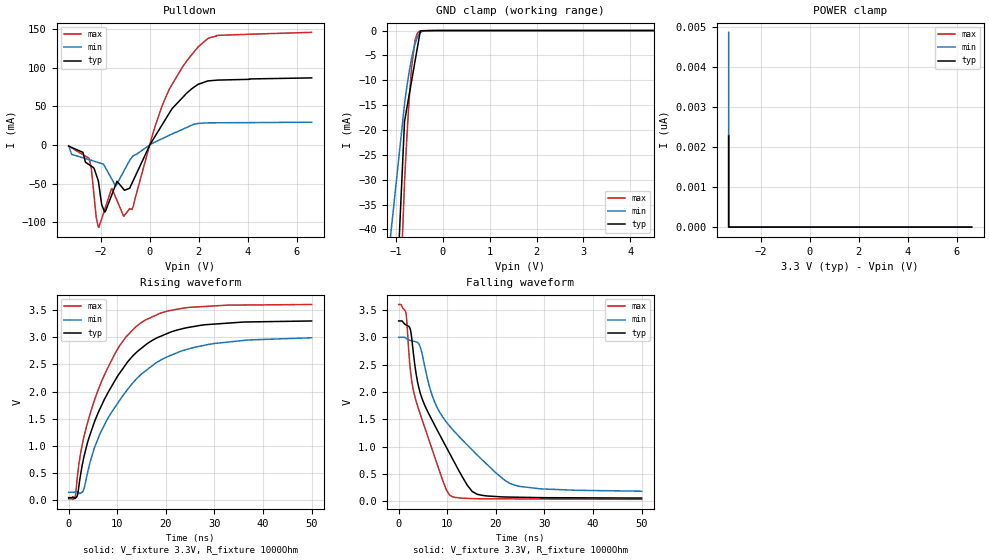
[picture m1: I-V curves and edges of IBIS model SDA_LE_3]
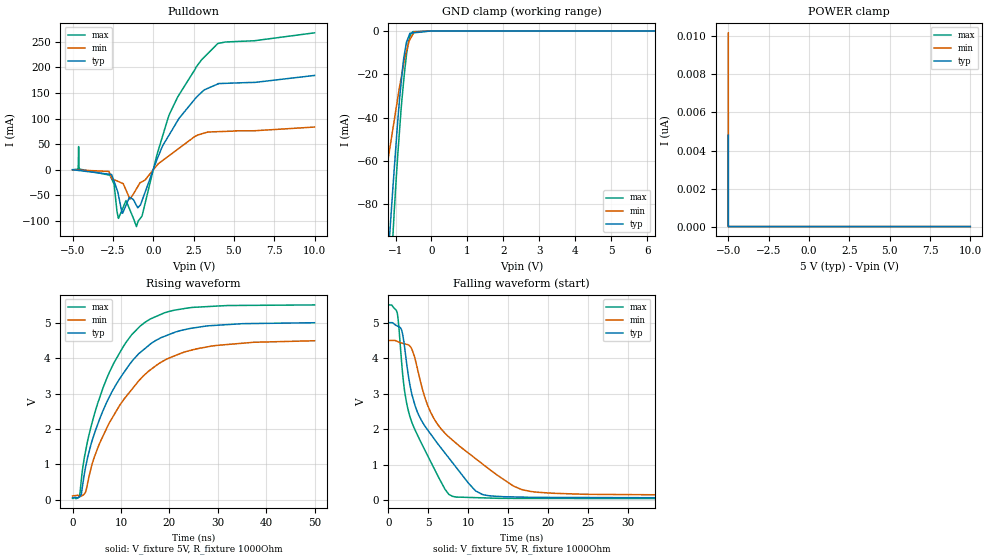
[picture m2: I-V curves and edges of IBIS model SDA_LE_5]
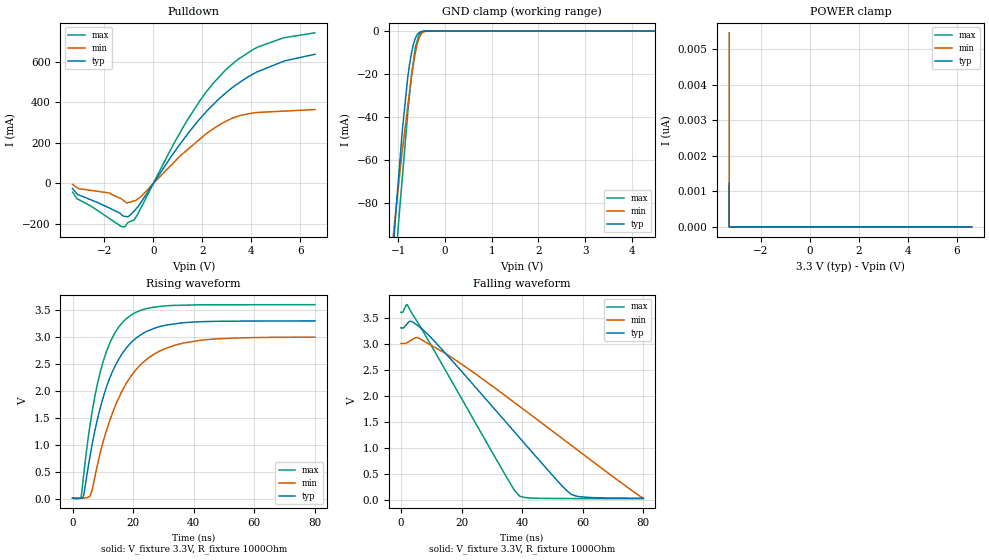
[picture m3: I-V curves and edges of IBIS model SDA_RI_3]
| Texas Instruments Incorporated
| Low-Power Bidirectional I2C Isolators
| Marketing part#   Voltage Range   Package-type   #pins/pkg drawing
| ISO1540D   3V-5.5V   SOIC   8-pin D
[IBIS Ver]   4.1
[File name]   iso1540.ibs
[File Rev]   1.0
[Date]   06/21/2012
[Source]   TIspiceD simulations
   Texas Instruments Incorporated.
   Analog eLab Design Center, HPA
   12500 TI Blvd
   Dallas, TX -75243
   For Support e-mail: elab_scm_ibis@list.ti.com
[Notes]   Revision History:
   Rev 1.0: 06/21/2012
   - C_comp although listed in numerical order of value are
   obtained from varying PVT conditions.
   For PVT conditions for each specific value, refer to the
   buffer description under respective [Model].
   IBIS model user is responsible for using appropriate
   C_comp to simulate for Signal Integrity.
   - IBIS model matched to TISPICED simulations
   - Pulldown data is non-monotonic, reflects circuit behavior
[Disclaimer] This model is designed as an aid for customers of Texas Instruments.
 TI and its licensors and suppliers make no warranties, either expressed
 or implied, with respect to this  model, including the warranties of
 merchantability or fitness for a particular purpose.
 The model is provided solely on an "as is" basis. The entire risk as to
 its quality and performance is with the customer.
[Copyright] (C)Copyright 2012 Texas Instruments Incorporated.
   All rights reserved.
|   Component ISO1540D
[Component]   ISO1540D
[Manufacturer]  Texas Instruments Incorporated
[Package]   |SOIC (D) 8-pin
|   typ   min   max
R_pkg   0.06626   0.03167   0.11324
L_pkg   2.49942nH   2.25405nH   2.79138nH
C_pkg   0.41610pF   0.38404pF   0.69535pF
[Pin]   signal_name   model_name   R_pin   L_pin   C_pin
1   VCC1   POWER   0.03718  2.27597n  0.43076p
2   SDA1   SDA_LE   0.09214  2.47816n  0.38404p
3   SCL1   SDA_LE   0.11324  2.79138n  0.40143p
4   GND1   GND   0.03348  2.51166n  0.69535p
5   GND2   GND   0.03167  2.53947n  0.67094p
6   SCL2   SDA_RI   0.09215  2.48718n  0.38609p
7   SDA2   SDA_RI   0.11323  2.77707n  0.39917p
8   VCC2   POWER   0.04038  2.25405n  0.46007p
[Model Selector] SDA_LE
SDA_LE_3   SDA I/O left side model for 3.0V - 3.6V
SDA_LE_5   SDA I/O left side model for 4.5V - 5.5V
[Model Selector] SDA_RI
SDA_RI_3   SDA I/O right side model for 3.0V - 3.6V
SDA_RI_5   SDA I/O right side model for 4.5V - 5.5V
| Models and submodels in the file (4): SDA_LE_3 (I/O_open_drain), SDA_LE_5 (I/O_open_drain), SDA_RI_3 (I/O_open_drain), SDA_RI_5 (I/O_open_drain)
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|   SDA Left 3.3V I/O Model
[Model]   SDA_LE_3
Model_type   I/O_open_drain
Polarity   Non-Inverting
Enable   Active-Low
Vinl = 0.5
Vinh = 2.52
Vmeas = 1.65
Vref = 1.65
Cref = 15pF
Rref = 1000
|   typ   min   max
|   (nom PVT)   (fast PVT)   (slow PVT)
C_comp   4.033p   3.367p   4.533p
|C_comp (High state)   4.033p   3.367p   4.533p
|C_comp (Low state)   5.596p   4.907p   5.983p
|PVT   Nom   Slow   Fast
[Voltage Range]   3.3   3   3.6
[Temperature Range]   27   136   -40
[Pullup Reference]   3.3   3   3.6
[Pulldown Reference]   -0   -0   -0
[Power Clamp Reference]   3.3   3   3.6
[GND Clamp Reference]   -0   -0   -0
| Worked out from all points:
|   slope of the pulldown table from 0 to 0.495 V, typ, clamps not added: 19.4 ohm
|   GND clamp passes 1 mA (typ) near -0.50 V on its own axis
|   falling waveform, V_fixture 3.3V, R_fixture 1000Ohm: 20-80 % time 8.4ns typ, 11.9ns min, 5.69ns max; typ from 3.3 V to 0.057 V
|   rising waveform, V_fixture 3.3V, R_fixture 1000Ohm: 20-80 % time 10.2ns typ, 12ns min, 8.59ns max; typ from 0.053 V to 3.3 V
[Pulldown]
|   Voltage   I(typ)   I(min)   I(max)
-3.3V     -1.441mA   -854.9uA   -1.481mA
-2.462V   -25.48mA   -19.01mA   -17.28mA
-2.095V   -46.15mA   -22.58mA   -105.6mA
-1.835V   -86.44mA   -27.36mA   -83.61mA
-1.533V   -63.51mA   -44.52mA   -56.4mA
-1.329V   -46.75mA   -49.98mA   -71.69mA
-1.058V   -57.16mA   -34.04mA   -92.04mA
-665.1mV  -45.59mA   -13.84mA   -78.65mA
800.2mV   41.16mA    12.55mA    72.1mA
1.984V    78.4mA     27.85mA    126.9mA
2.741V    83.72mA    28.65mA    141.4mA
6.6V      86.64mA    29.42mA    145.4mA
[GND Clamp]
|   Voltage   I(typ)   I(min)   I(max)
-3.3V     -815.4mA   -640mA     -971mA
-1.208V   -99.67mA   -49.74mA   -133.4mA
-1.091V   -75.48mA   -39.34mA   -97.6mA
-816.4mV  -18.3mA    -14.78mA   -30.7mA
-780mV    -16.34mA   -12.22mA   -23.92mA
-720.5mV  -13.12mA   -8.521mA   -14.39mA
-665.1mV  -10.12mA   -5.641mA   -7.366mA
-591.4mV  -6.144mA   -2.677mA   -1.944mA
-551.3mV  -3.973mA   -1.563mA   -734.8uA
-478.8mV  -55.54uA   -412.4uA   -98.93uA
-198.6mV  -17.66uA   -327nA     -154.7nA
6.6V      0A         0A         0A
[POWER Clamp]
|   Voltage   I(typ)   I(min)   I(max)
-3.3V     2.274nA    4.859nA    2.297nA
-3.3V     0A         0A         0A
-3.3V     0A         0A         0A
6.6V      0A         0A         0A
[Ramp]
R_load = 1000
|   typ   min   max
dV/dt_r   1.94673/1.02316e-08   1.70302/1.18334e-08   2.14001/8.58161e-09
dV/dt_f   1.9456/8.391e-09   1.69022/1.18691e-08   2.13948/5.67055e-09
[Falling Waveform]
V_fixture = 3.3V
V_fixture_min = 3V
V_fixture_max = 3.6V
R_fixture = 1000Ohm
C_fixture = 0F
|   Time   V(typ)   V(min)   V(max)
0s        3.3V       3V         3.6V
1.498ns   3.229V     2.986V     3.446V
2.486ns   3.108V     2.942V     2.34V
3.414ns   2.436V     2.921V     1.888V
5.316ns   1.765V     2.49V      1.361V
7.433ns   1.387V     1.809V     805.8mV
10.44ns   882.6mV    1.38V      115.5mV
15.14ns   177.9mV    938.5mV    48mV
23.88ns   73.47mV    293.4mV    42.9mV
50ns      57.34mV    183mV      34.2mV
[Rising Waveform]
V_fixture = 3.3V
V_fixture_min = 3V
V_fixture_max = 3.6V
R_fixture = 1000Ohm
C_fixture = 0F
|   Time   V(typ)   V(min)   V(max)
0s        52.63mV    150.1mV    32.79mV
1.366ns   41.87mV    157.1mV    77.54mV
1.856ns   113mV      153.4mV    486.1mV
2.88ns    687.9mV    157.4mV    1.06V
6.136ns   1.625V     1.156V     2.046V
9.812ns   2.245V     1.751V     2.744V
13.76ns   2.704V     2.214V     3.185V
18.88ns   3.014V     2.576V     3.44V
25.88ns   3.197V     2.813V     3.552V
50ns      3.297V     2.988V     3.599V
|   SDA Left 5V I/O Model
[Model]   SDA_LE_5
Model_type   I/O_open_drain
Polarity   Non-Inverting
Enable   Active-Low
Vinl = 0.5
Vinh = 3.85
Vmeas = 2.5
Vref = 2.5
Cref = 15pF
Rref = 1000
|   typ   min   max
|   (nom PVT)   (fast PVT)   (slow PVT)
C_comp   3.824p   3.201p   4.341p
|C_comp (ON state)   3.824p   3.201p   4.341p
|C_comp (OFF state)   4.090p   3.369p   4.747p
|PVT   Nom   Slow   Fast
[Voltage Range]   5   4.5   5.5
[Temperature Range]   27   136   -40
[Pullup Reference]   5   4.5   5.5
[Pulldown Reference]   -0   -0   -0
[Power Clamp Reference]   5   4.5   5.5
[GND Clamp Reference]   -0   -0   -0
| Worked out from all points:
|   slope of the pulldown table from 0 to 0.75 V, typ, clamps not added: 13.5 ohm
|   GND clamp passes 1 mA (typ) near -0.59 V on its own axis
|   falling waveform, V_fixture 5V, R_fixture 1000Ohm: 20-80 % time 5.86ns typ, 8.17ns min, 3.71ns max; typ from 5 V to 0.061 V
|   rising waveform, V_fixture 5V, R_fixture 1000Ohm: 20-80 % time 10ns typ, 11.6ns min, 8.51ns max; typ from 0.058 V to 5 V
[Pulldown]
|   Voltage   I(typ)   I(min)   I(max)
-5V       114.9uA    34.82uA    189.2uA
-4.66V    -1.19mA    -456.2uA   1.163mA
-4.624V   -1.328mA   -507.9uA   45.41mA
-4.584V   -1.482mA   -565.8uA   1.547mA
-2.677V   -8.802mA   -8.11mA    -10.73mA
-2.169V   -47.15mA   -22.82mA   -93.81mA
-1.93V    -84.92mA   -26.14mA   -78.43mA
-1.686V   -69.33mA   -39.6mA    -60.1mA
-1.039V   -69.58mA   -37.18mA   -111mA
1.024V    70.1mA     28.52mA    109.9mA
2.995V    151.3mA    70.22mA    214.8mA
10V       184.4mA    83.55mA    267.7mA
[GND Clamp]
|   Voltage   I(typ)   I(min)   I(max)
-5V       -1.078A    -841.4mA   -1.257A
-1.536V   -182.6mA   -122mA     -238.4mA
-1.234V   -111.6mA   -63.88mA   -147.4mA
-1.215V   -106.8mA   -60.09mA   -141mA
-1.108V   -80.87mA   -48.84mA   -105.3mA
-1.073V   -72.38mA   -45.15mA   -94.57mA
-911.4mV  -36.12mA   -28.15mA   -51.25mA
-767.8mV  -12.11mA   -14.79mA   -22.09mA
-695.2mV  -5.155mA   -9.331mA   -10.98mA
-638.6mV  -2.707mA   -5.775mA   -4.887mA
-516.2mV  -876.4uA   -1.491mA   -277.5uA
10V       0A         0A         0A
[POWER Clamp]
|   Voltage   I(typ)   I(min)   I(max)
-5V       4.793nA    10.19nA    5.967nA
-5V       0A         0A         0A
-5V       0A         0A         0A
10V       0A         0A         0A
[Ramp]
R_load = 1000
|   typ   min   max
dV/dt_r   2.96373/1.0022e-08   2.62546/1.15746e-08   3.27428/8.51231e-09
dV/dt_f   2.96329/5.82536e-09   2.62267/8.14594e-09   3.2739/3.70478e-09
[Falling Waveform]
V_fixture = 5V
V_fixture_min = 4.5V
V_fixture_max = 5.5V
R_fixture = 1000Ohm
C_fixture = 0F
|   Time   V(typ)   V(min)   V(max)
0s        5V         4.5V       5.5V
1.116ns   4.906V     4.473V     5.271V
1.99ns    4.392V     4.406V     3.159V
2.813ns   3.125V     4.308V     2.279V
3.802ns   2.399V     3.552V     1.764V
5.274ns   1.872V     2.489V     1.1V
8.039ns   1.056V     1.693V     109.3mV
11.79ns   160.4mV    1.021V     67.6mV
17.66ns   83.02mV    252.6mV    51.97mV
50ns      61.18mV    128.9mV    43.5mV
[Rising Waveform]
V_fixture = 5V
V_fixture_min = 4.5V
V_fixture_max = 5.5V
R_fixture = 1000Ohm
C_fixture = 0F
|   Time   V(typ)   V(min)   V(max)
0s        57.65mV    113mV      42.31mV
1.449ns   85.7mV     109.5mV    119.9mV
3.02ns    1.136V     406.6mV    1.605V
4.453ns   1.844V     1.19V      2.385V
6.324ns   2.525V     1.81V      3.171V
10.37ns   3.545V     2.791V     4.298V
13.98ns   4.158V     3.402V     4.904V
18.66ns   4.596V     3.913V     5.257V
25.66ns   4.864V     4.262V     5.436V
50ns      4.997V     4.489V     5.499V
|   SDA Right 3.3V I/O Model
[Model]   SDA_RI_3
Model_type   I/O_open_drain
Polarity   Non-Inverting
Enable   Active-Low
Vinl = 0.9
Vinh = 2.52
Vmeas = 1.65
Vref = 1.65
Cref = 15pF
Rref = 1000
|   typ   min   max
|   (nom PVT)   (fast PVT)   (slow PVT)
C_comp   1.957p   1.640p   2.653p
|C_comp (ON state)   1.957p   1.640p   2.653p
|C_comp (OFF state)   4.105p   3.069p   5.182p
|PVT   Nom   Slow   Fast
[Voltage Range]   3.3   3   3.6
[Temperature Range]   27   136   -40
[Pullup Reference]   3.3   3   3.6
[Pulldown Reference]   -0   -0   -0
[Power Clamp Reference]   3.3   3   3.6
[GND Clamp Reference]   -0   -0   -0
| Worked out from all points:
|   slope of the pulldown table from 0 to 0.495 V, typ, clamps not added: 5.5 ohm
|   GND clamp passes 1 mA (typ) near -0.56 V on its own axis
|   falling waveform, V_fixture 3.3V, R_fixture 1000Ohm: 20-80 % time 29.5ns typ, 41ns min, 21.1ns max; typ from 3.3 V to 0.023 V
|   rising waveform, V_fixture 3.3V, R_fixture 1000Ohm: 20-80 % time 10.4ns typ, 12.9ns min, 8.02ns max; typ from 0.018 V to 3.3 V
[Pulldown]
|   Voltage   I(typ)   I(min)   I(max)
-3.3V     -25.45mA   -4.956mA   -43.12mA
-3.115V   -52.44mA   -21.31mA   -76.35mA
-1.778V   -122.9mA   -47.71mA   -174.6mA
-1.163V   -162.6mA   -89.49mA   -214.4mA
-1.026V   -164.4mA   -94.36mA   -191.6mA
-629.9mV  -115.6mA   -76.18mA   -150.1mA
1.395V    243.6mA    166.8mA    313.9mA
2.16V     353.6mA    245.2mA    451.2mA
2.925V    442.8mA    304.5mA    556.7mA
4.271V    551.8mA    350.1mA    672.8mA
5.31V     602.1mA    356.5mA    718.1mA
6.6V      637.1mA    364.5mA    742.8mA
[GND Clamp]
|   Voltage   I(typ)   I(min)   I(max)
-3.3V     -759.2mA   -570.2mA   -927.9mA
-1.142V   -112.7mA   -103.6mA   -137.6mA
-1.078V   -93.5mA    -89.71mA   -115.2mA
-1.002V   -71.26mA   -74.08mA   -92.05mA
-909.3mV  -46.13mA   -55.48mA   -68.05mA
-794.9mV  -21.68mA   -35.16mA   -38.3mA
-755.4mV  -15.47mA   -28.13mA   -29.6mA
-709.8mV  -9.809mA   -20.52mA   -19.87mA
-629.9mV  -3.29mA    -9.977mA   -7.425mA
-524.4mV  -338uA     -1.998mA   -1.07mA
-327.3mV  -31.85uA   -19.07uA   -2.263uA
6.6V      0A         0A         0A
[POWER Clamp]
|   Voltage   I(typ)   I(min)   I(max)
-3.3V     1.227nA    5.456nA    1.121nA
-3.3V     0A         0A         0A
-3.3V     0A         0A         0A
6.6V      0A         0A         0A
[Ramp]
R_load = 1000
|   typ   min   max
dV/dt_r   1.96937/1.04301e-08   1.78574/1.29228e-08   2.15107/8.02123e-09
dV/dt_f   1.96592/2.94956e-08   1.78636/4.10048e-08   2.15033/2.1068e-08
[Falling Waveform]
V_fixture = 3.3V
V_fixture_min = 3V
V_fixture_max = 3.6V
R_fixture = 1000Ohm
C_fixture = 0F
|   Time   V(typ)   V(min)   V(max)
0s        3.3V       3V         3.6V
2.053ns   3.378V     3.016V     3.746V
3.441ns   3.425V     3.067V     3.6V
5.125ns   3.363V     3.115V     3.444V
6.988ns   3.279V     3.067V     3.264V
17.59ns   2.624V     2.699V     2.19V
34.49ns   1.5V       1.995V     467.7mV
39.29ns   1.179V     1.786V     61.85mV
56.27ns   98.33mV    1.04V      18.34mV
80ns      23.47mV    22.8mV     16.12mV
[Rising Waveform]
V_fixture = 3.3V
V_fixture_min = 3V
V_fixture_max = 3.6V
R_fixture = 1000Ohm
C_fixture = 0F
|   Time   V(typ)   V(min)   V(max)
0s        17.61mV    22.73mV    14.85mV
2.821ns   15.93mV    17.82mV    39.79mV
3.672ns   72.41mV    19.96mV    452mV
5.796ns   807mV      56.5mV     1.385V
10.04ns   1.871V     1.051V     2.537V
13.91ns   2.448V     1.698V     3.072V
18.49ns   2.846V     2.209V     3.376V
25.53ns   3.129V     2.633V     3.54V
36.73ns   3.266V     2.891V     3.59V
80ns      3.3V       2.999V     3.6V
